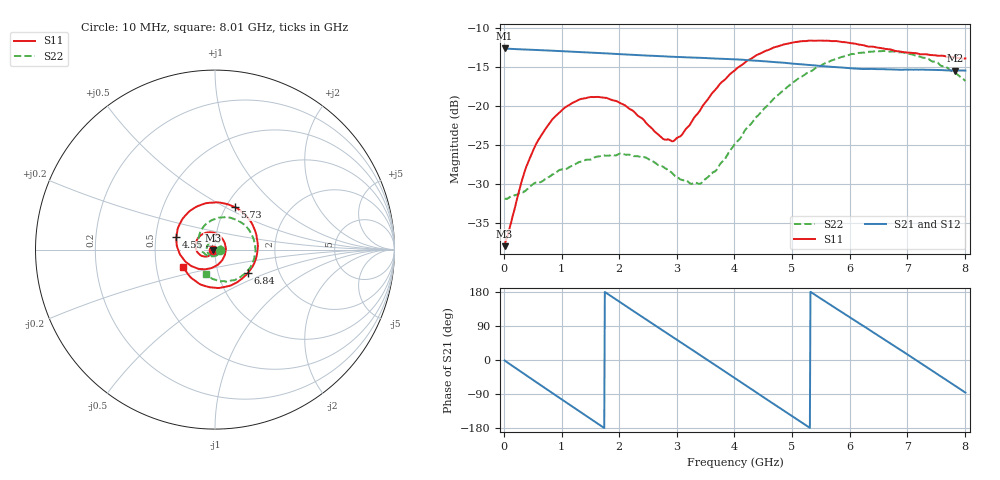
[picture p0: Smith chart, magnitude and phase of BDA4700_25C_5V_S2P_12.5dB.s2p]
!Agilent Technologies,E5071B,MY42404982,A.09.10
!Date: Mon Oct 20 13:32:23 2025
!Data & Calibration Information:
!Freq	S11:SOLT2(ON)	S21:SOLT2(ON)	S12:SOLT2(ON)	S22:SOLT2(ON)
# Hz S RI R 50
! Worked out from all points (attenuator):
!   801 points, 10 MHz to 8.01 GHz, reference 50 ohm
!   highest |S21| = -12.61 dB at 10 MHz (marker M1); lowest = -15.5 dB at 7.83 GHz (marker M2)
!   lowest |S11| = -38.0 dB at 10 MHz (marker M3), VSWR 1.03, Z = 48.8 - j0.165 ohm
!   |S11| at or under -10 dB: start of sweep to end of sweep
!   |S22| runs from -32.0 to -12.9 dB; largest |S21 - S12| = 0.0018
!   S11 on the Smith chart (normalised r, x): 10 MHz: 0.98, -0.00; 4.55 GHz: 0.64, +0.09; 5.73 GHz: 1.10, +0.56; 6.84 GHz: 1.38, -0.38; 8.01 GHz: 0.69, -0.14
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1e7  -0.0124 -0.00169  0.2342 -0.00505  0.2341 -0.00536  0.0253 -0.00101
3.5e8  -0.0245 -0.0277  0.1847 -0.1381  0.1845 -0.1381  0.0216 -0.0179
5.7e8  -0.0435 -0.0386  0.116 -0.1972  0.1158 -0.1973  0.0134 -0.0293
8.8e8  -0.0783 -0.0331  -0.00573 -0.226  -0.00586 -0.2262  -0.00972 -0.0356
1.35e9  -0.1091 0.0211  -0.1692 -0.1434  -0.1692 -0.1436  -0.0417 -0.0139
1.94e9  -0.0546 0.0929  -0.2031 0.0733  -0.2032 0.0733  -0.0317 0.0361
2.33e9  0.0122 0.0852  -0.1085 0.1821  -0.1085 0.1822  0.000793 0.0474
2.68e9  0.0539 0.0371  0.016 0.2085  0.0159 0.2085  0.0272 0.0314
2.96e9  0.0569 -0.0191  0.1109 0.1743  0.111 0.1742  0.0346 0.00911
3.4e9  -0.000747 -0.0931  0.1983 0.0471  0.1984 0.047  0.0165 -0.0269
3.69e9  -0.0702 -0.1091  0.1939 -0.0547  0.1939 -0.0553  -0.0116 -0.037
4.01e9  -0.1506 -0.0782  0.1329 -0.1484  0.1331 -0.1482  -0.0487 -0.0294
4.55e9  -0.2156 0.0694  -0.0428 -0.1885  -0.0426 -0.1886  -0.0908 0.0389
4.98e9  -0.1539 0.2021  -0.1554 -0.1048  -0.1557 -0.1053  -0.0708 0.1184
5.35e9  -0.0343 0.2604  -0.1824 0.00966  -0.1826 0.00913  -0.00396 0.1686
5.73e9  0.1088 0.2374  -0.135 0.1158  -0.1349 0.1159  0.0919 0.1756
6.21e9  0.2257 0.0991  -0.00785 0.1725  -0.00646 0.1729  0.1974 0.0975
6.68e9  0.2173 -0.0791  0.1184 0.1243  0.1187 0.1243  0.2212 -0.0315
6.84e9  0.1823 -0.1313  0.1469 0.0875  0.1476 0.0866  0.2081 -0.0755
7.33e9  0.0219 -0.2136  0.1625 -0.0523  0.1626 -0.0527  0.1134 -0.1685
7.83e9  -0.1411 -0.1487  0.064 -0.1561  0.0638 -0.1564  -0.0142 -0.1631
8.01e9  -0.1767 -0.0976  0.0114 -0.1684  0.0117 -0.1686  -0.0506 -0.1354
